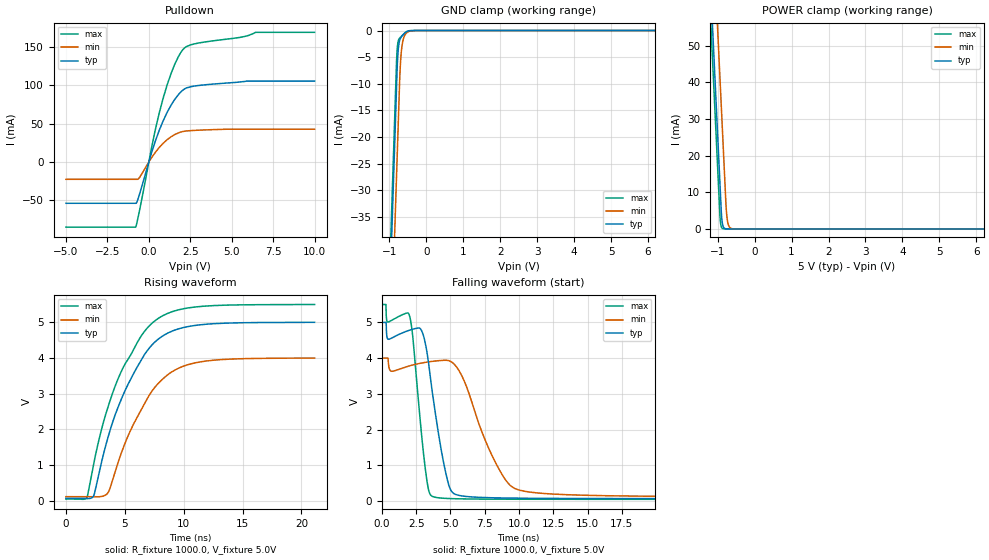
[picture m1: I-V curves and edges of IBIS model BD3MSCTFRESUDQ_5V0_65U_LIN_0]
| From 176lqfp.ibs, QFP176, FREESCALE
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[Model] BD3MSCTFRESUDQ_5V0_65U_LIN_0
Model_type I/O_open_drain
Polarity   Non-Inverting
Enable   Active-High
| var   typ   min   max
C_comp   2.47005pF  2.46580pF  2.47120pF
Vinl = 1.4V
Vinh = 3.575V
Vmeas = 2.5V
Cref  = 50.0pF
Rref  = 1.0kOhm
Vref  = 5.0V
[Model Spec]
Vinl 1.75000V 1.40000V 1.92500V
Vinh 3.25000V 2.60000V 3.57500V
| variable   typ   min   max
[Temperature Range] 25.0 150.0 -40.0
| variable   typ   min   max
[Voltage Range] 5.0V 4.0V 5.5V
| variable   typ   min   max
[POWER Clamp Reference] 5.0V 4.0V 5.5V
| variable   typ   min   max
[GND Clamp Reference] 0V 0V 0V
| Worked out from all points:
|   slope of the pulldown table from 0 to 0.75 V, typ, clamps not added: 15.8 ohm
|   GND clamp passes 1 mA (typ) near -0.65 V on its own axis
|   POWER clamp passes 1 mA (typ) near -0.86 V on its own axis
|   rising waveform, R_fixture 1000.0, V_fixture 5.0V: 20-80 % time 3.51ns typ, 3.41ns min, 3.6ns max; typ from 0.066 V to 5 V
|   falling waveform, R_fixture 1000.0, V_fixture 5.0V: 20-80 % time 1.16ns typ, 2.39ns min, 791ps max; typ from 5 V to 0.066 V
[POWER Clamp]
-5V       875.6mA    904.4mA    866.6mA
-1.24V    76.57mA    105.4mA    67.61mA
-1.16V    59.57mA    88.38mA    50.61mA
-1.09V    44.69mA    73.5mA     35.73mA
-1.01V    27.69mA    56.5mA     18.73mA
-930mV    10.69mA    39.5mA     2.356mA
-890mV    2.973mA    31mA       332.6uA
-860mV    935uA      24.63mA    82.04uA
-780mV    47.58uA    7.63mA     8.877uA
-750mV    18.44uA    3.369mA    7.12uA
-610mV    3.063uA    76.44uA    3.683uA
10V       0A         0A         0A
[GND Clamp]
-5V       -902.4mA   -919mA     -897.5mA
-1.01V    -54.49mA   -71.14mA   -49.58mA
-810mV    -11.99mA   -28.64mA   -7.082mA
-800mV    -9.863mA   -26.52mA   -5.134mA
-780mV    -5.991mA   -22.27mA   -2.957mA
-750mV    -3.059mA   -15.89mA   -1.788mA
-720mV    -1.885mA   -9.515mA   -1.426mA
-700mV    -1.501mA   -6.433mA   -1.281mA
-680mV    -1.249mA   -4.428mA   -1.146mA
-610mV    -677.8uA   -1.367mA   -660.7uA
-490mV    -100.9uA   -235.7uA   -82.78uA
10V       923.5pA    10.55nA    924.7pA
| variable   typ   min   max
[Pullup Reference] 5.0V 4.0V 5.5V
| variable   typ   min   max
[Pulldown Reference] 0V 0V 0V
[Pullup]
-5V       0A         0A         0A
0V        0A         0A         0A
10V       0A         0A         0A
[Pulldown]
-5V       -53.66mA   -22.48mA   -84.7mA
-790mV    -53.66mA   -22.48mA   -84.33mA
-540mV    -40.34mA   -19.48mA   -60.85mA
390mV     27.06mA    12.51mA    41.86mA
860mV     53.35mA    24.25mA    82.68mA
1.57V     81.59mA    35.75mA    127.3mA
1.92V     90.84mA    38.9mA     142.1mA
2.18V     95.33mA    40.13mA    148.8mA
3.21V     100mA      41.59mA    155.5mA
5.55V     104.2mA    42.7mA     162.3mA
6.44V     105.2mA    42.7mA     168.6mA
10V       105.2mA    42.7mA     168.6mA
[Ramp]
dV/dt_r 2.9602V/3.51087ns 2.33196V/3.41373ns 3.2717V/3.5981ns
dV/dt_f 2.96036V/1.16298ns 2.32971V/2.38912ns 3.27185V/791.14701ps
R_load = 1000.0
| Removed startup time: 0s 0s 0s  .
| Removed end time: 21.1ns.
[Rising Waveform]
R_fixture   = 1000.0
V_fixture   = 5.0V
V_fixture_min = 4.0V
V_fixture_max = 5.5V
0s        65.95mV    112.7mV    46.91mV
1.78ns    59.35mV    112.7mV    89.24mV
2.39ns    165.8mV    112.5mV    1.091V
3.53ns    1.73V      205.8mV    2.581V
5.21ns    3.219V     1.765V     3.931V
6.49ns    4V         2.601V     4.665V
7.55ns    4.446V     3.178V     5.042V
9.23ns    4.781V     3.657V     5.32V
11.36ns   4.929V     3.889V     5.443V
21.12ns   5V         3.999V     5.5V
| Removed startup time: 0s 0s 0s  .
| Removed end time: 27.28ns.
[Falling Waveform]
R_fixture   = 1000.0
V_fixture   = 5.0V
V_fixture_min = 4.0V
V_fixture_max = 5.5V
0s        5V         4V         5.5V
465ps     4.527V     3.898V     5.008V
2.04ns    4.784V     3.786V     5.148V
2.965ns   4.705V     3.867V     1.574V
3.66ns    3.09V      3.908V     133.5mV
4.705ns   703.1mV    3.939V     72.15mV
5.41ns    179.7mV    3.767V     62.8mV
8.115ns   89.87mV    1.205V     51.54mV
9.77ns    79.47mV    338.2mV    49.42mV
27.29ns   66.06mV    117.1mV    46.92mV
